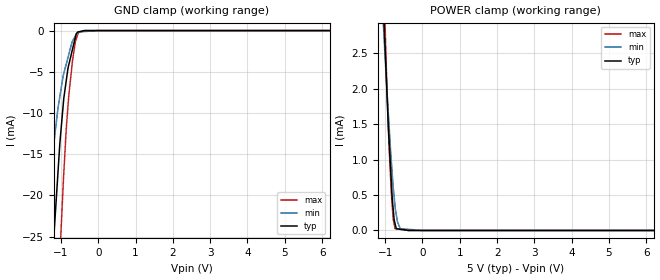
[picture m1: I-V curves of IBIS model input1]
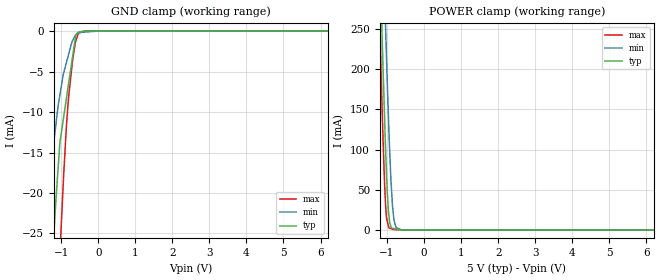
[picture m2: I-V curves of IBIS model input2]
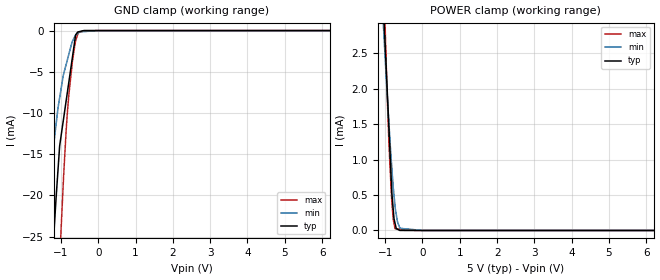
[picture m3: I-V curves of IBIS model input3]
| Texas Instruments Incorporated
| ADS126x Precision, 6-Channel and 11-Channel, 40-kSPS, 24-Bit, Delta-Sigma,
| Analog-to-Digital Converters With Programmable Gain Amplifier
| and Voltage Reference
[IBIS Ver]   4.1
[File name]   ads1261.ibs
[File Rev]   1.1
[Date]   03/23/2018
[Source]
| Texas Instruments Incorporated.
| Analog-eLab Design Center, HPA
| 12500 TI Blvd
| Dallas, TX -75243
[Notes]   Revision History:
| Rev 1.1: 03/23/2018
| - Updated models for AIN5, AIN4, AIN1 and AIN0
| Rev 1.0: 02/15/2018
| - Initial version of the model
| - Model generated from simulations in SPECTRE
| - C_comp although listed in numerical order of value are
|   obtained from varying PVT conditions. For PVT conditions for
|   each specific value refer the buffer description under
|   respective [Model]. IBIS model user is responsible for using
|   appropriate C_comp to simulate for Signal Integrity.
| - Warnings regarding combined Non-monotonicity of various models
|   have been reviewed and considered minor and can be ignored.
[Disclaimer]
| This model is designed as an aid for customers of Texas Instruments.
| TI and its licensors and suppliers make no warranties, either expressed
| or implied, with respect to this  model, including the warranties of
| merchantability or fitness for a particular purpose. The model is
| provided solely on an "as is" basis. The entire risk as to its quality
| and performance is with the customer.
| This model is subject to change without notice. Texas Instruments
| Incorporated is not responsible for updating this model.
[Copyright]
 (C) Copyright 2018 Texas Instruments Incorporated. All rights reserved.
|  Component ADS1261 32-pin VQFN - RHB Package
|  Part # ADS1261
[Component]   ADS1261
[Manufacturer]   TI
[Package]   |32 VQFN
|   typ   min   max
R_pkg   0.1   0.08   0.12
L_pkg   1.0nH   0.8nH   1.2nH
C_pkg   0.2pF   0.16pF   0.24pF
[Pin]   signal_name   model_name   R_pin   L_pin   C_pin
1   AINCOM   nc   NA   NA   NA
2   CAPP   nc   NA   NA   NA
3   CAPN   nc   NA   NA   NA
4   AVDD   power   NA   NA   NA
5   AVSS   gnd   NA   NA   NA
6   REFOUT   nc   NA   NA   NA
7   _PWDN   input1   NA   NA   NA
8   _RESET   input1   NA   NA   NA
9   START   input2   NA   NA   NA
10   _CS   input2   NA   NA   NA
11   SCLK   input2   NA   NA   NA
12   DIN   input2   NA   NA   NA
13   _DRDY   output1   NA   NA   NA
14   DOUT/_DRDY   output2   NA   NA   NA
15   BYPASS   nc   NA   NA   NA
16   DGND   gnd   NA   NA   NA
17   DVDD   power   NA   NA   NA
18   CLKIN   input3   NA   NA   NA
19   NC   nc   NA   NA   NA
20   NC   nc   NA   NA   NA
21   NC   nc   NA   NA   NA
22   NC   nc   NA   NA   NA
23   AIN9   nc   NA   NA   NA
24   AIN8   nc   NA   NA   NA
25   AIN7   nc   NA   NA   NA
26   AIN6   nc   NA   NA   NA
27   AIN5   io   NA   NA   NA
28   AIN4   io   NA   NA   NA
29   AIN3   io   NA   NA   NA
30   AIN2   io   NA   NA   NA
31   AIN1   nc   NA   NA   NA
32   AIN0   nc   NA   NA   NA
| Models and submodels in the file (6): input1 (Input), input2 (Input), input3 (Input), io (I/O), output1 (Output), output2 (3-state)
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|   input1 Model
[Model]   input1
Model_type   Input
Vinl = 1.5
Vinh = 3.5
|   typ   min   max
C_comp   2.097pF   1.769pF   2.332pF
|  Where Nom  PVT is Nominal Process,   5V,  27C
|   Fast PVT is Strong Process,   5.25V, -40C
|   Slow PVT is Weak Process,   2.7V, 135C
[Model spec]
|subparameter
Vinl   1.500   0.810   1.575
Vinh   3.500   1.890   3.675
[Voltage Range]   5   2.7   5.25
|Junction Temperature
[Temperature Range]   27   135   -40
[Power Clamp Reference]   5   2.7   5.25
[GND Clamp Reference]   0   0   0
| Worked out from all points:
|   GND clamp passes 1 mA (typ) near -0.62 V on its own axis
|   POWER clamp passes 1 mA (typ) near -0.87 V on its own axis
[GND Clamp]
|   Voltage   I(typ)   I(min)   I(max)
-5V       -411.9mA   -286.8mA   -505.9mA
-1.431V   -44.29mA   -24.6mA    -72.55mA
-1.25V    -29.13mA   -15.99mA   -51.34mA
-1.125V   -20.36mA   -11.14mA   -37.39mA
-1.02V    -13.12mA   -7.699mA   -26.27mA
-925.5mV  -8.237mA   -5.215mA   -17.34mA
-859.4mV  -6.098mA   -4.079mA   -11.96mA
-791mV    -4.157mA   -2.903mA   -7.903mA
-691.6mV  -2.279mA   -1.289mA   -3.661mA
-613mV    -793.6uA   -632.4uA   -1.318mA
-552.1mV  -174.7uA   -320.7uA   -465.3uA
10V       0A         0A         0A
[POWER Clamp]
|   Voltage   I(typ)   I(min)   I(max)
-5V       83.73mA    65.22mA    101.9mA
-1.066V   3.562mA    3.079mA    4.189mA
-1.03V    2.953mA    2.734mA    3.452mA
-1.003V   2.596mA    2.462mA    2.902mA
-895.1mV  1.272mA    1.477mA    1.176mA
-834.1mV  673.8uA    972.1uA    517.1uA
-785.2mV  299.6uA    615.8uA    163.3uA
-736.6mV  99.9uA     351.5uA    25.61uA
-671.1mV  23.45uA    123.9uA    21uA
-592.2mV  17.25uA    24.58uA    15.44uA
-136uV    0A         0A         0A
10V       0A         0A         0A
|   input2 Model
[Model]   input2
Model_type   Input
Vinl = 1.5
Vinh = 3.5
|   typ   min   max
C_comp   2.031pF   1.769pF   2.237pF
|  Where Nom  PVT is Nominal Process,   5V,  27C
|   Fast PVT is Strong Process,   5.25V, -40C
|   Slow PVT is Weak Process,   2.7V, 135C
[Model spec]
|subparameter
Vinl   1.500   0.810   1.575
Vinh   3.500   1.890   3.675
[Voltage Range]   5   2.7   5.25
|Junction Temperature
[Temperature Range]   27   135   -40
[Power Clamp Reference]   5   2.7   5.25
[GND Clamp Reference]   0   0   0
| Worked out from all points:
|   GND clamp passes 1 mA (typ) near -0.62 V on its own axis
|   POWER clamp passes 1 mA (typ) near -0.73 V on its own axis
[GND Clamp]
|   Voltage   I(typ)   I(min)   I(max)
-5V       -410mA     -285.3mA   -503.9mA
-1.44V    -44.59mA   -24.64mA   -73.15mA
-1.25V    -28.81mA   -15.66mA   -50.96mA
-1.136V   -20.34mA   -11.26mA   -38.24mA
-1.021V   -13.29mA   -7.467mA   -26.02mA
-861.5mV  -8.371mA   -3.915mA   -11.87mA
-793.7mV  -6.276mA   -2.755mA   -7.859mA
-694.3mV  -3.203mA   -1.183mA   -3.67mA
-607.1mV  -510.3uA   -447uA     -1.215mA
-553.2mV  -173.2uA   -262uA     -464.5uA
-368.8mV  -2.276uA   -122.5uA   -967.2nA
10V       0A         0A         0A
[POWER Clamp]
|   Voltage   I(typ)   I(min)   I(max)
-5V       7.793A     7.929A     7.725A
-1.25V    441.2mA    609.4mA    349.1mA
-1.15V    269.3mA    433.6mA    177.9mA
-1.14V    252.9mA    417.7mA    161.7mA
-1.067V   141.2mA    296mA      58.5mA
-1.036V   94.04mA    246.8mA    28.32mA
-962.5mV  23.07mA    140.7mA    4.923mA
-896.4mV  4.471mA    63.13mA    1.697mA
-821.5mV  1.806mA    16.35mA    431.7uA
-757.8mV  1.269mA    3.093mA    388.9uA
-607.2mV  1.677uA    49.97uA    287.8uA
10V       0A         0A         0A
|   input3 Model
[Model]   input3
Model_type   Input
Vinl = 1.5
Vinh = 3.5
|   typ   min   max
C_comp   2.088pF   1.785pF   2.310pF
|  Where Nom  PVT is Nominal Process,   5V,  27C
|   Fast PVT is Strong Process,   5.25V, -40C
|   Slow PVT is Weak Process,   2.7V, 135C
[Model spec]
|subparameter
Vinl   1.500   0.810   1.575
Vinh   3.500   1.890   3.675
[Voltage Range]   5   2.7   5.25
|Junction Temperature
[Temperature Range]   27   135   -40
[Power Clamp Reference]   5   2.7   5.25
[GND Clamp Reference]   0   0   0
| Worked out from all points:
|   GND clamp passes 1 mA (typ) near -0.62 V on its own axis
|   POWER clamp passes 1 mA (typ) near -0.86 V on its own axis
[GND Clamp]
|   Voltage   I(typ)   I(min)   I(max)
-5V       -411.9mA   -286.8mA   -505.9mA
-1.431V   -44.3mA    -24.61mA   -72.57mA
-1.25V    -29.13mA   -15.99mA   -51.34mA
-1.136V   -20.62mA   -11.56mA   -38.61mA
-1.02V    -13.49mA   -7.699mA   -26.27mA
-940.2mV  -10.99mA   -5.469mA   -18.67mA
-859.7mV  -8.464mA   -4.084mA   -11.98mA
-791.3mV  -6.315mA   -2.908mA   -7.918mA
-691.6mV  -3.18mA    -1.281mA   -3.661mA
-607.2mV  -526.9uA   -539.8uA   -1.237mA
-552.1mV  -174.7uA   -334.3uA   -465.3uA
10V       0A         0A         0A
[POWER Clamp]
|   Voltage   I(typ)   I(min)   I(max)
-5V       83.73mA    65.22mA    101.9mA
-1.066V   3.518mA    3.079mA    4.189mA
-1.036V   3.031mA    2.785mA    3.575mA
-1.003V   2.647mA    2.462mA    2.902mA
-950.8mV  2.04mA     1.964mA    1.972mA
-895.1mV  1.391mA    1.477mA    1.176mA
-821.5mV  531.1uA    879.8uA    407.7uA
-785.2mV  302.4uA    615.8uA    163.3uA
-736.6mV  104.6uA    351.5uA    25.62uA
-671.1mV  17.6uA     123.9uA    22.61uA
-607.2mV  809.2nA    34.72uA    19.67uA
10V       0A         0A         0A
